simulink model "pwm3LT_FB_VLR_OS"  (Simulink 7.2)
settings: Solver=ode3  SolverMode=SingleTasking  StartTime=0.0  StopTime=0.1  FixedStep=10e-6  MaxStep=1e-4  RelTol=1e-3
libraries: PE_CONV_OS x1

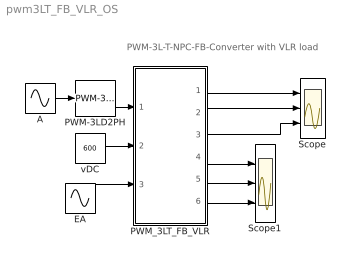
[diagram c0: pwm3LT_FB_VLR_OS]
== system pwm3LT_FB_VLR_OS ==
  note: PWM-3L-T-NPC-FB-Converter with VLR load
  A : Sin  Amplitude=.8  Frequency=2*pi*50  Phase=[0 ]  SampleTime=0
  EA : Sin  Amplitude=0  Frequency=2*pi*50  Phase=[0 ]  SampleTime=0
  PWM-3LD2PH : PE_CONV_OS/Converter_Control/PWM-3LD2PH  SystemSampleTime=-1  FT=900  PHT=0  A=0.5  O1=0.5  O2=-0.5  DT=1e-6
  PWM_3LT_FB_VLR : Subsystem  mask(pwm_3LT_FB_VLR_OS){RL=1, LL=1e-3}
      mask prompts: RL "Load Resistance"; LL "Load Inductance"
      mask help: Open Source 3-Level T-NPC Full Bridge Converter Input Vector u: u[0]= L3L1_TD1.gate u[1]= L3L1_TD2.gate u[2]= L3L1_TD3.gate u[3]= L3L1_TD4.gate u[4]= L3L2_TD1.gate u[5]= L3L2_TD2.gate u[6]= L3L2_TD3.gate u[7]= L3L2_TD4.gate u[8]= VDC u[9]= EL Output Vector y: y[0]= Va.v, Output AC Voltage to middle point y[1]= Ia.I, Output AC Current y[2]= Vab.V, Output AC Voltage y[3]= T1.I y[4]= D1.I y[5]= T1.V y[6]= T2.I y[7]= D2.I y[8]= T2.V y[9]= D5.I y[10]= D5.V y[11]= IDC1, Input DC Current y[12]= IDC2, Input DC Current Parameter Vector p: p[0]=RL p[1]=LL You can pause the simulation during running, cha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
  Scope : Scope  NumInputPorts=3
  Scope1 : Scope  NumInputPorts=3
  vDC : Constant  Value=600  OutDataType=sfix(16)  OutScaling=2^0
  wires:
  A/1 -> PWM-3LD2PH/1
  PWM_3LT_FB_VLR/4("iT1, iD1,vT1") -> Scope1/1
  PWM_3LT_FB_VLR/5("iT2, iD2,vT2") -> Scope1/2
  PWM_3LT_FB_VLR/6("iDC1, iDC2") -> Scope1/3
  PWM_3LT_FB_VLR/1(vA) -> Scope/1
  EA/1 -> PWM_3LT_FB_VLR/3(E_A)
  vDC/1 -> PWM_3LT_FB_VLR/2(vDC)
  PWM-3LD2PH/1 -> PWM_3LT_FB_VLR/1(Sw)
  PWM_3LT_FB_VLR/2(iA) -> Scope/2
  PWM_3LT_FB_VLR/3(vAB) -> Scope/3

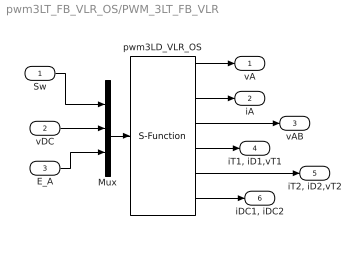
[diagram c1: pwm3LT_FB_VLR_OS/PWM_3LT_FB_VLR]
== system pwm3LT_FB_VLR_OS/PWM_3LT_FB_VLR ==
  Sw : Inport  OutDataType=sfix(16)  OutScaling=2^0
  vDC : Inport  Port=2  OutDataType=sfix(16)  OutScaling=2^0
  E_A : Inport  Port=3  OutDataType=sfix(16)  OutScaling=2^0
  Mux : Mux  Inputs="[8  1  1]"
  pwm3LD_VLR_OS : S-Function  FunctionName=s_pwm_3LT_FB_VLR_OS  Parameters="[RL  LL]"  EnableBusSupport=off
  vA : Outport  OutDataType=sfix(16)  OutScaling=2^0
  iA : Outport  Port=2  OutDataType=sfix(16)  OutScaling=2^0
  vAB : Outport  Port=3  OutDataType=sfix(16)  OutScaling=2^0
  "iT1, iD1,vT1" : Outport  Port=4  OutDataType=sfix(16)  OutScaling=2^0
  "iT2, iD2,vT2" : Outport  Port=5  OutDataType=sfix(16)  OutScaling=2^0
  "iDC1, iDC2" : Outport  Port=6  OutDataType=sfix(16)  OutScaling=2^0
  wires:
  pwm3LD_VLR_OS/5 -> "iT2, iD2,vT2"/1
  pwm3LD_VLR_OS/4 -> "iT1, iD1,vT1"/1
  pwm3LD_VLR_OS/3 -> vAB/1
  pwm3LD_VLR_OS/2 -> iA/1
  pwm3LD_VLR_OS/1 -> vA/1
  E_A/1 -> Mux/3
  Mux/1 -> pwm3LD_VLR_OS/1
  vDC/1 -> Mux/2
  Sw/1 -> Mux/1
  pwm3LD_VLR_OS/6 -> "iDC1, iDC2"/1
